(* Logix 5000 DataType export PF_Safety_Monitor_Diagnostics; software revision 32.01 *)

TYPE PF_Safety_Monitor_Diagnostics :
STRUCT
   NA : SINT;
   NA1 : SINT;
   NA2 : SINT;
   Status : SINT;   // Bit 0=Mode(0-config, 1=protect) Bit 4 Status S12 Bit 5 Status S21 Bit 6 Status S32 Bit 7 Status S41
   OSSD_2_1 : SINT;
   OSSD_4_3 : SINT;
   OSSD_6_5 : SINT;
   OSSD_8_7 : SINT;
   OSSD_10_9 : SINT;
   OSSD_12_11 : SINT;
   OSSD_14_13 : SINT;
   OSSD_16_15 : SINT;
   Device_Index_Present : SINT[32];   // Indexes that are present from 0 to 255
   Device_Index_Color : SINT[128];   // Two Indexes per byte, bits 0-3 device 1, bits 4-7 device 2
END_STRUCT
END_TYPE
